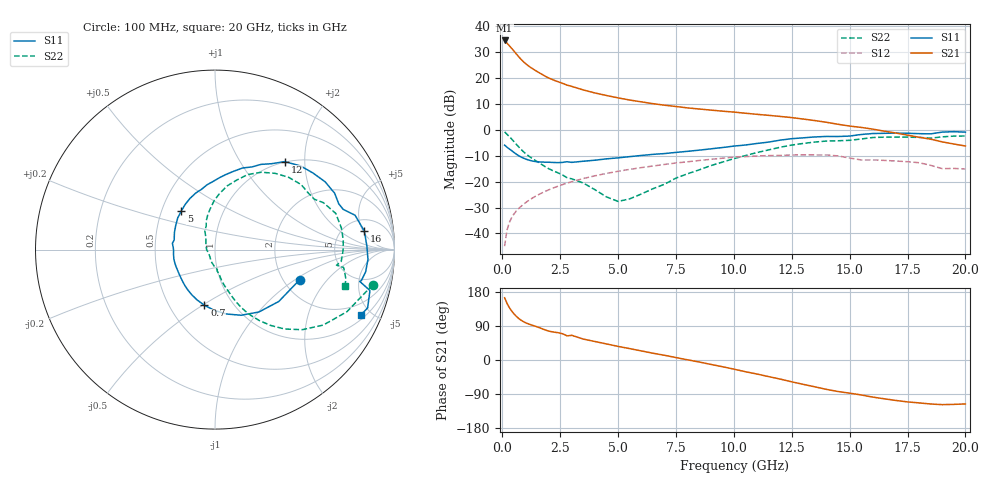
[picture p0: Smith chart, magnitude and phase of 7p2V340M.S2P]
! Infineon Technologies  Discrete & RF Semiconductors
! bfp620
! VCE =  2.3 V,  IC =  40 mA
! Common Emitter S-Parameters:  Sep 2002
# GHz  S  MA  R  50
!  f  S11  S21  S12  S22
! GHz  MAG  ANG  MAG  ANG  MAG  ANG  MAG  ANG
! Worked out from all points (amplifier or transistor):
!   59 points, 100 MHz to 20 GHz, reference 50 ohm
!   highest |S21| = 34.3 dB at 100 MHz (marker M1)
!   |S21| within 3 dB of that: start of sweep to 400.9 MHz
!   unconditionally stable (mu >= 1): 2.671 GHz to 9.846 GHz; 17.19 GHz to end of sweep
!   at 1 GHz: K = 0.83, MSG = 26.8 dB, |S12| = -28.2 dB
!   at 5.5 GHz: K = 1.04, MAG = 12.1 dB, |S12| = -15.3 dB
!   at 20 GHz: K = 1.25, MAG = 1.4 dB, |S12| = -15.2 dB
!   S11 on the Smith chart (normalised r, x): 100 MHz: 2.44, -1.09; 700 MHz: 0.74, -0.51; 5 GHz: 0.63, +0.30; 12 GHz: 0.99, +1.60; 16 GHz: 7.70, +5.30; 20 GHz: 1.23, -4.35
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0.1  0.501 -19.5  51.8 164.3  0.0057 63.5  0.9 -12.6
0.2  0.4581 -39.1  46.04 150.0  0.0114 66.1  0.8127 -25.2
0.3  0.4251 -54.9  41.21 138.7  0.0161 65.7  0.7351 -34.9
0.4  0.3937 -68.3  36.71 129.6  0.02 64.8  0.6603 -42.5
0.5  0.3639 -80.2  32.51 122.1  0.0236 64.0  0.5892 -48.7
0.6  0.3376 -91.0  28.72 115.6  0.0269 63.4  0.5244 -53.7
0.7  0.3156 -100.8  25.45 110.1  0.03 62.9  0.4675 -57.9
0.8  0.2978 -109.5  22.7 105.4  0.033 62.5  0.4193 -61.3
1  0.2717 -123.6  18.64 98.4  0.039 62.0  0.3464 -66.0
1.2  0.2543 -134.5  15.93 93.7  0.045 61.5  0.2966 -69.0
1.6  0.2379 -152.3  12.35 85.4  0.057 59.8  0.2275 -73.4
2.2  0.2327 -173.3  9 73.8  0.0751 56.2  0.1602 -79.0
2.8  0.2401 171.6  7.153 63.7  0.0932 51.7  0.1182 -84.7
3.5  0.2456 157.0  5.773 55.2  0.1142 45.7  0.0935 -92.3
5  0.2856 131.1  4.067 35.9  0.1574 32.0  0.0414 -145.1
7  0.3447 102.4  2.942 12.5  0.2128 13.2  0.0884 125.4
10.5  0.5039 66.0  2.06 -30.9  0.3019 -25.8  0.3154 85.1
12  0.6256 51.6  1.789 -50.3  0.317 -43.3  0.4566 66.4
13.5  0.7206 31.6  1.488 -70.8  0.3249 -62.1  0.5745 44.6
16  0.8386 7.0  1.019 -97.9  0.2605 -86.2  0.7023 16.7
17  0.854 -3.7  0.857 -106.8  0.2479 -94.2  0.7167 4.2
20  0.8908 -24.1  0.482 -116.0  0.1743 -103.7  0.7515 -15.7
